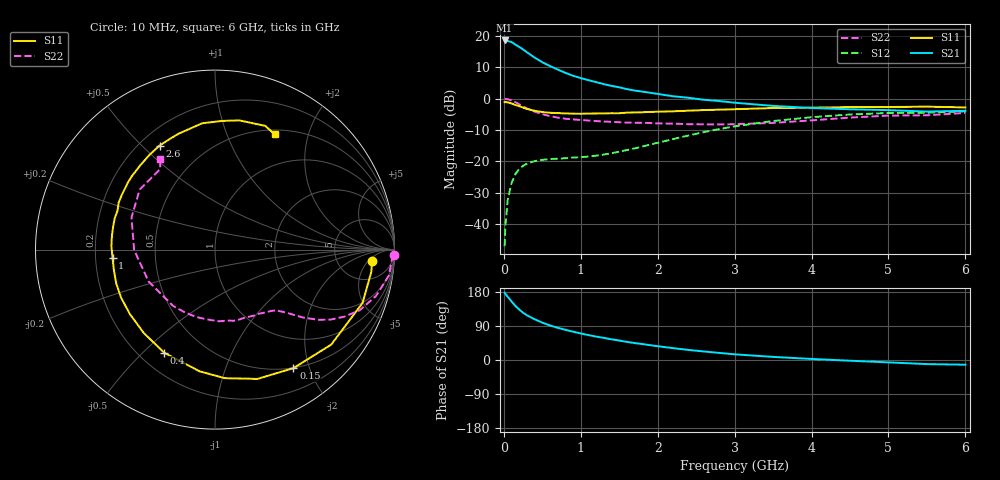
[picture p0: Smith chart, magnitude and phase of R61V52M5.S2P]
! SIEMENS Small Signal Semiconductors
! BFR193
! Si NPN RF Bipolar Junction Transistor in SOT23
! VCE = 1.5 V  IC = 2.5 mA
! Common Emitter S-Parameters:  May  1996
# GHz  S  MA  R  50
!  f  S11  S21  S12  S22
! GHz  MAG  ANG  MAG  ANG  MAG  ANG  MAG  ANG
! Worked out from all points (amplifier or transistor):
!   36 points, 10 MHz to 6 GHz, reference 50 ohm
!   highest |S21| = 18.5 dB at 10 MHz (marker M1)
!   |S21| within 3 dB of that: start of sweep to 257.9 MHz
!   unconditionally stable (mu >= 1): 1.083 GHz to 2.082 GHz
!   at 250 MHz: K = 0.27, MSG = 18.5 dB, |S12| = -21.4 dB
!   at 1.4 GHz: K = 1.11, MAG = 8.7 dB, |S12| = -17.4 dB
!   at 6 GHz: K = 1.00, MSG = 0.1 dB, |S12| = -4.0 dB
!   S11 on the Smith chart (normalised r, x): 10 MHz: 12, -7; 150 MHz: 0.50, -1.75; 400 MHz: 0.30, -0.58; 1 GHz: 0.27, -0.04; 2.6 GHz: 0.28, +0.57; 6 GHz: 0.55, +1.50
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0.01  0.8773 -4.2  8.399 177.7  0.0045 84.7  0.9958 -1.7
0.02  0.8799 -8.0  8.376 174.5  0.0094 86.5  0.9868 -3.4
0.05  0.8742 -19.9  8.238 166.9  0.0243 79.4  0.9794 -8.5
0.1  0.8362 -39.3  7.915 154.5  0.0454 69.4  0.9333 -16.1
0.15  0.7919 -56.5  7.232 142.7  0.0629 61.2  0.8736 -22.8
0.2  0.7584 -71.8  6.63 133.3  0.0764 54.3  0.812 -27.4
0.25  0.7183 -85.7  6.044 124.7  0.0854 48.8  0.7509 -31.3
0.3  0.6836 -97.2  5.449 118.0  0.0922 44.7  0.6975 -34.1
0.4  0.6406 -116.2  4.489 107.6  0.1014 39.0  0.6213 -37.6
0.5  0.6109 -130.6  3.78 98.6  0.1062 36.0  0.5659 -39.8
0.6  0.5947 -143.1  3.29 91.2  0.1093 34.9  0.5256 -41.7
0.7  0.5878 -153.1  2.897 85.0  0.1107 34.8  0.4985 -43.5
0.8  0.5818 -161.1  2.563 79.7  0.1128 35.5  0.4778 -45.2
1  0.5728 -175.4  2.117 70.0  0.117 38.6  0.4567 -49.0
1.1  0.5775 178.0  1.962 65.8  0.1198 41.0  0.4479 -51.5
1.6  0.5972 153.9  1.413 47.8  0.1519 53.3  0.4152 -65.3
2.2  0.6277 131.5  1.088 31.3  0.2269 58.7  0.3999 -87.1
2.6  0.6564 118.1  0.958 22.5  0.2927 56.1  0.3896 -105.5
3.5  0.7074 95.8  0.765 8.2  0.44 41.4  0.4104 -154.4
4.5  0.7327 79.3  0.676 -1.9  0.5586 21.9  0.4984 159.0
5.5  0.7442 67.9  0.622 -10.8  0.595 3.8  0.5428 124.3
6  0.7234 62.7  0.639 -12.4  0.6289 -1.3  0.5913 120.9
